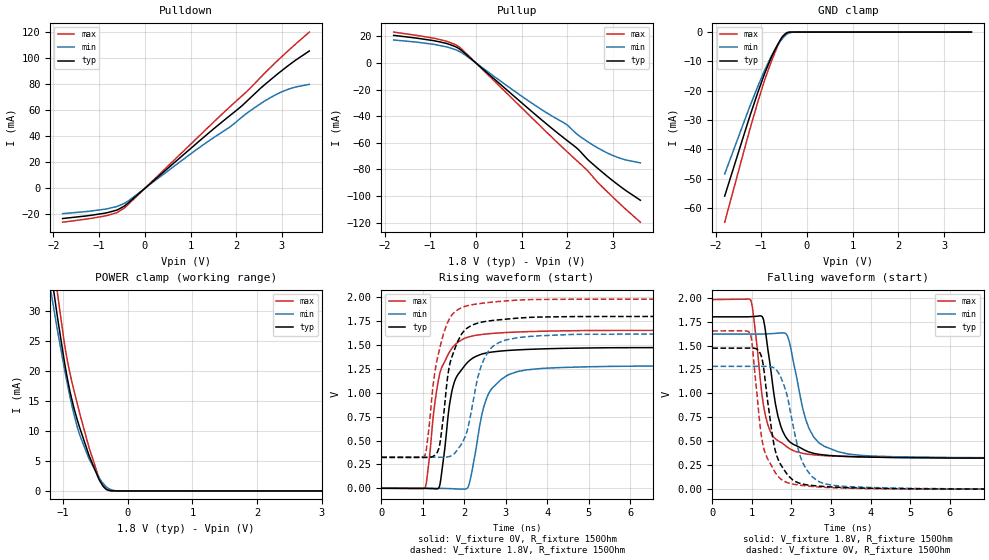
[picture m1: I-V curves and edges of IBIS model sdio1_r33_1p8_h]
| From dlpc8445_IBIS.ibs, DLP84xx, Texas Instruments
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|**********************  Begin SDIO *************************************
|   r33_1p8_h
[Model]   sdio1_r33_1p8_h
Model_type   I/O
Polarity   Non-Inverting
Enable   Active-High
Vinl = 0
Vinh = 0.8
Vmeas = 0.9
Vref = 1.8
Cref = 2pF
Rref = 100000
|   typ   min   max
C_comp   4.069pF   3.633pF   4.416pF
[Voltage Range]   1.8   1.62   1.98
[Temperature Range]   27   150   -40
[Pullup Reference]   1.8   1.62   1.98
[Pulldown Reference]   0   0   0
[Power Clamp Reference]   1.8   1.62   1.98
[GND Clamp Reference]   0   0   0
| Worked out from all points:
|   slope of the pulldown table from 0 to 0.27 V, typ, clamps not added: 32.7 ohm
|   slope of the pullup table from 0 to 0.27 V, typ, clamps not added: 33.3 ohm
|   GND clamp passes 1 mA (typ) near -0.50 V on its own axis
|   POWER clamp passes 1 mA (typ) near -0.39 V on its own axis
|   falling waveform, V_fixture 1.8V, R_fixture 150Ohm: 20-80 % time 378ps typ, 475ps min, 331ps max; typ from 1.8 V to 0.323 V
|   rising waveform, V_fixture 0V, R_fixture 150Ohm: 20-80 % time 336ps typ, 417ps min, 362ps max; typ from 0 V to 1.47 V
|   rising waveform, V_fixture 1.8V, R_fixture 150Ohm: 20-80 % time 353ps typ, 429ps min, 368ps max; typ from 0.323 V to 1.8 V
|   falling waveform, V_fixture 0V, R_fixture 150Ohm: 20-80 % time 357ps typ, 454ps min, 331ps max; typ from 1.47 V to 0 V
[Pulldown]
|   Voltage   I(typ)   I(min)   I(max)
-1.8V     -23.11mA   -19.37mA   -25.9mA
-822.6mV  -18.62mA   -15.6mA    -20.75mA
-595.8mV  -16.39mA   -13.67mA   -18.29mA
-450mV    -13.58mA   -11.51mA   -15.11mA
1.289V    39.16mA    33.63mA    43.47mA
1.856V    55.57mA    46.88mA    62.25mA
2.12V     63.09mA    54.44mA    70.66mA
2.266V    67.88mA    58.41mA    75.26mA
2.531V    76.61mA    64.84mA    84.87mA
2.855V    86.16mA    71.54mA    96.18mA
3.13V     93.77mA    75.79mA    105.2mA
3.6V      105.2mA    79.66mA    119.7mA
[GND Clamp]
|   Voltage   I(typ)   I(min)   I(max)
-1.8V     -55.9mA    -48.35mA   -64.79mA
-1.282V   -30.22mA   -26.65mA   -34.97mA
-1.103V   -21.87mA   -19.59mA   -25.31mA
-946.8mV  -15.01mA   -13.77mA   -17.35mA
-790.2mV  -8.997mA   -8.533mA   -10.48mA
-622.8mV  -3.762mA   -4.011mA   -4.146mA
-541.8mV  -1.721mA   -2.298mA   -1.694mA
-450mV    -362.9uA   -857.5uA   -222.8uA
-347.4mV  -20.24uA   -138.5uA   -4.035uA
-234mV    -328.9nA   -10.21uA   -105nA
3.6V      0A         0A         0A
[Pullup]
|   Voltage   I(typ)   I(min)   I(max)
-1.8V     20.73mA    17.25mA    23.19mA
-882mV    16.48mA    13.74mA    18.29mA
-622.8mV  14.45mA    11.89mA    16.11mA
-363.6mV  10.6mA     8.667mA    11.98mA
1.138V    -33.96mA   -28.22mA   -38.27mA
1.969V    -57.56mA   -45.96mA   -65.85mA
2.201V    -63.78mA   -53.19mA   -73.2mA
2.434V    -72.09mA   -58.91mA   -80.52mA
2.639V    -78.39mA   -63.33mA   -88.72mA
2.871V    -85.06mA   -67.59mA   -96.66mA
3.13V     -92.06mA   -71.29mA   -105.2mA
3.6V      -103.2mA   -75.08mA   -119.7mA
[POWER Clamp]
|   Voltage   I(typ)   I(min)   I(max)
-1.8V     86.44mA    75.43mA    99.9mA
-1.238V   40.27mA    36.32mA    46.12mA
-1.109V   30.39mA    27.98mA    34.62mA
-1.082V   28.41mA    26.29mA    32.35mA
-941.4mV  19.05mA    18.09mA    22mA
-838.8mV  13.99mA    12.97mA    16.93mA
-741.6mV  10.42mA    9.224mA    12.8mA
-595.8mV  5.776mA    5.267mA    7.057mA
-450mV    2.018mA    2.285mA    2.309mA
-320.4mV  226.3uA    591.6uA    146.1uA
-126mV    319.1nA    8.169uA    136.9nA
3.6V      0A         0A         0A
[Ramp]
R_load = 150
|   typ   min   max
dV/dt_r   0.883531/3.34876e-10   0.769179/4.16731e-10   0.991643/3.61511e-10
dV/dt_f   0.886304/3.77292e-10   0.776574/4.69395e-10   0.992029/3.30749e-10
[Falling Waveform]
V_fixture = 1.8V
V_fixture_min = 1.62V
V_fixture_max = 1.98V
R_fixture = 150Ohm
C_fixture = 0F
|   Time   V(typ)   V(min)   V(max)
0s        1.8V       1.62V      1.98V
975ps     1.802V     1.62V      1.97V
1.265ns   1.799V     1.62V      953mV
1.44ns    1.356V     1.623V     628.8mV
1.655ns   766.4mV    1.629V     506.7mV
1.885ns   527.1mV    1.611V     442.3mV
2.095ns   458.8mV    1.238V     394.9mV
2.455ns   386.7mV    624.5mV    363.3mV
3.18ns    346.1mV    391.2mV    343.7mV
10ns      322.7mV    325.3mV    326.5mV
[Rising Waveform]
V_fixture = 0V
V_fixture_min = 0V
V_fixture_max = 0V
R_fixture = 150Ohm
C_fixture = 0F
|   Time   V(typ)   V(min)   V(max)
0s        229.9uV    586.7uV    145.6uV
1.055ns   -1.232mV   414.7uV    5.836mV
1.385ns   3.598mV    -511.3uV   1.152V
1.7ns     1.014V     -4.005mV   1.464V
2.02ns    1.289V     -7.988mV   1.571V
2.115ns   1.333V     39.99mV    1.585V
2.415ns   1.404V     756.2mV    1.609V
2.545ns   1.417V     951.5mV    1.615V
3.07ns    1.443V     1.189V     1.631V
10ns      1.473V     1.283V     1.653V
[Rising Waveform]
V_fixture = 1.8V
V_fixture_min = 1.62V
V_fixture_max = 1.98V
R_fixture = 150Ohm
C_fixture = 0F
|   Time   V(typ)   V(min)   V(max)
0s        322.7mV    325.3mV    326.5mV
1.05ns    322.1mV    325.1mV    343.2mV
1.345ns   374.5mV    324.6mV    1.348V
1.425ns   505.3mV    324.7mV    1.496V
1.65ns    1.299V     333.5mV    1.78V
2ns       1.65V      520.1mV    1.901V
2.325ns   1.728V     1.16V      1.93V
2.47ns    1.743V     1.346V     1.938V
2.995ns   1.769V     1.551V     1.96V
10ns      1.8V       1.62V      1.98V
[Falling Waveform]
|Gnd
V_fixture = 0V
V_fixture_min = 0V
V_fixture_max = 0V
R_fixture = 150Ohm
C_fixture = 0F
|   Time   V(typ)   V(min)   V(max)
0s        1.473V     1.283V     1.653V
950ps     1.474V     1.283V     1.63V
1.01ns    1.474V     1.283V     1.496V
1.19ns    1.433V     1.283V     721.7mV
1.315ns   1.205V     1.283V     403.9mV
1.565ns   448.3mV    1.265V     191mV
1.875ns   164.8mV    1.001V     71.56mV
2.265ns   55.1mV     293.6mV    39.19mV
2.815ns   28.17mV    59.25mV    19.71mV
10ns      229.9uV    587.1uV    145.7uV
